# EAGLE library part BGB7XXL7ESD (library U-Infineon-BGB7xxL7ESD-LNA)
High Performance LNAs BGB707L7ESD 0.05 - 10 GHz Operational Bandwidth NFmin = 0.60 dB at 2.4 GHz Source: Datasheet BGB741L7ESD 0.03 - 5 GHz Operational Bandwidth NFmin = 1.05 dB at 2.4 GHz Source: Datasheet
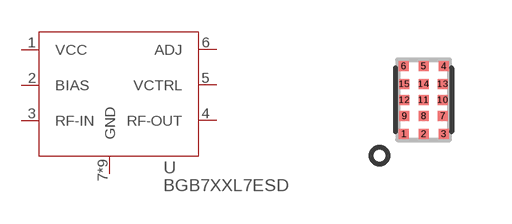
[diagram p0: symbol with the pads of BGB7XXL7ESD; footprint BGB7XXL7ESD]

Designator prefix U

## BGB7XXL7ESD  [BGB7XXL7ESD]
1  VCC  pwr
2  BIAS
3  RF-IN  in
4  RF-OUT  out
5  VCTRL  in
6  ADJ  pwr
7  GND  pwr
8  GND  pwr
9  GND  pwr
10  GND  pwr
11  GND  pwr
12  GND  pwr
13  GND  pwr
14  GND  pwr
15  GND  pwr

## Footprint BGB7XXL7ESD (pad centres in mm)
smd 0.25 x 0.25: 1 -0.5,-0.85; 2 0,-0.85; 3 0.5,-0.85; 4 0.5,0.85; 5 0,0.85; 6 -0.5,0.85; 7 0.48,-0.4; 8 0,-0.4; 9 -0.48,-0.4; 10 0.48,0; 11 0,0; 12 -0.48,0; 13 0.48,0.4; 14 0,0.4; 15 -0.48,0.4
